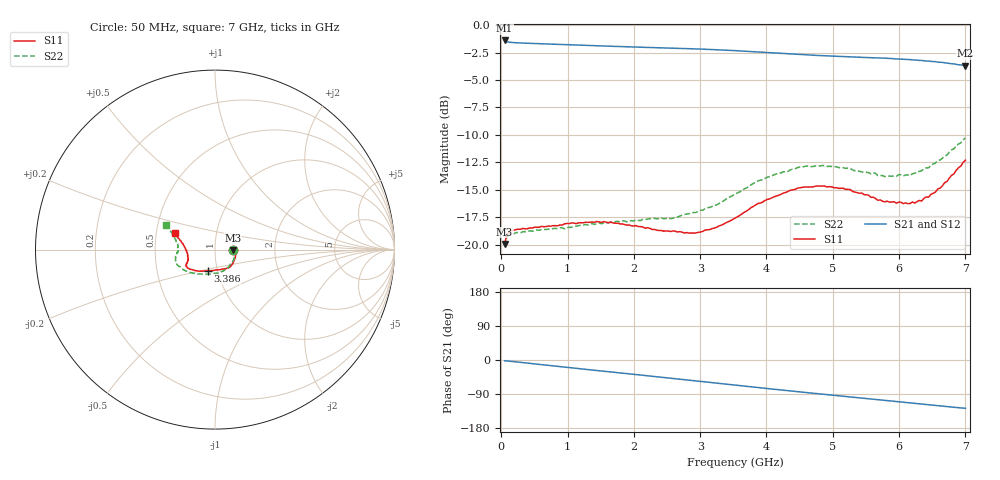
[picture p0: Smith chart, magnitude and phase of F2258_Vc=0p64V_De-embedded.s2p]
! Integrated Device Technology
! Corporate Headquarters
! 6024 Silver Creek Valley Road
! San Jose, CA 95138  USA
! Phone:  1-408-284-8200
! Toll Free:  1-800-223-1366
! Webpage:  http://www.idt.com/
! Timing and RF Division
! 515 Groton Road, Suite 102
! Westford, MA 01886-6024
! Device:  F2258
! Description: Voltage Variable RF Attenuator
! Frequency:  50.0 -  6000.00 MHz
! Package:  3x3 mm Thin QFN Plastic Package: 16 pin
! Ports:  2 RF, 2 DC
!  Pin  1  = NC
!  Pin  2  = NC
!  Pin  3  = RF2  = Port 2
!  Pin  4  = GND
!  Pin  5  = Vdd
!  Pin  6  = NC
!  Pin  7  = VCTRL
!  Pin  8  = NC
!  Pin  9  = GND
!  Pin 10  = RF1  = Port 1
!  Pin 11  = NC
!  Pin 12  = NC
!  Pin 13  = NC
!  Pin 14  = NC
!  Pin 15  = NC
!  Pin 16  = NC
! Vcntrl:  0.640 Volts
! Vdd:  +3.300 Volts
! Current:  1.113 mA
! Data:  The device was measured on a the F2258 evaluation board which has
!  individual transmission lines to the RF pins.  Data was collected
!  using a calibrated network analyzer.  The evaluation board was
!  de-embedded using a TRL calibration technique.
!  The reference plane is the edge of the package pin.
! Misc:  SN 10
!  Action Tracker AT0285
! Date Measured:  2014-12-10
! Date:  2016-01-13  MJV
! Note:
!  Integrated Device Technology supplies this data as a sample of measured
!  data at the package pin for this product.  Your particular data for this
!  product may vary.
!  Data was taken at 25 degrees C.
!  Integrated Device Technology reserves the right to change this data at anytime.
!Freq_(GHz)  S11M_(dB)  S11P_(deg)  S21M_(dB)  S21P_(deg)  S12M_(dB)  S12P_(deg)  S22M_(dB)  S22P_(deg)
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# GHz S dB R 50
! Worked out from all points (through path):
!   201 points, 50 MHz to 7 GHz, reference 50 ohm
!   highest |S21| = -1.40 dB at 50 MHz (marker M1); lowest = -3.7 dB at 7 GHz (marker M2)
!   group delay of S21, straight-line fit = 50.5 ps
!   lowest |S11| = -19.9 dB at 50 MHz (marker M3), VSWR 1.22, Z = 61.2 - j0.498 ohm
!   |S11| at or under -10 dB: start of sweep to end of sweep
!   |S22| runs from -20.1 to -10.3 dB; largest |S21 - S12| = 0.00097
!   S11 on the Smith chart (normalised r, x): 50 MHz: 1.22, -0.01; 3.386 GHz: 0.90, -0.22; 7 GHz: 0.62, +0.12
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0.05  -19.91 -2.3  -1.40 -2.0  -1.40 -2.0  -20.12 -2.7
0.08475  -19.06 -3.7  -1.51 -2.5  -1.51 -2.5  -19.31 -4.3
0.15425  -18.68 -6.0  -1.58 -3.7  -1.58 -3.7  -18.99 -7.5
0.71025  -18.28 -25.7  -1.72 -14.2  -1.72 -14.2  -18.57 -31.3
1.2315  -18.00 -42.8  -1.83 -23.9  -1.83 -23.9  -18.21 -53.0
1.6485  -17.92 -52.4  -1.93 -31.5  -1.92 -31.5  -17.94 -66.0
2.37825  -18.70 -68.7  -2.06 -44.8  -2.06 -44.8  -17.61 -85.3
2.58675  -18.73 -74.6  -2.10 -48.6  -2.10 -48.6  -17.59 -91.9
2.93425  -18.92 -88.4  -2.17 -55.1  -2.17 -55.1  -17.06 -104.3
3.386  -17.99 -109.3  -2.28 -63.7  -2.29 -63.7  -15.85 -122.7
3.525  -17.57 -115.3  -2.33 -66.3  -2.33 -66.3  -15.41 -127.9
4.0115  -15.87 -133.6  -2.50 -75.3  -2.50 -75.3  -13.84 -144.6
4.46325  -14.85 -144.1  -2.67 -83.5  -2.67 -83.5  -12.98 -156.5
4.7065  -14.72 -147.5  -2.74 -87.8  -2.75 -87.8  -12.87 -161.1
5.2625  -14.96 -153.8  -2.90 -97.4  -2.91 -97.4  -13.03 -169.9
5.64475  -15.78 -158.9  -2.99 -104.0  -2.99 -104.0  -13.49 -175.8
5.6795  -15.94 -158.8  -2.98 -104.6  -2.99 -104.6  -13.70 -176.0
5.85325  -16.11 -162.8  -3.04 -107.7  -3.05 -107.7  -13.74 179.3
6.166  -16.24 -171.0  -3.14 -113.3  -3.15 -113.2  -13.69 172.8
6.33975  -16.02 -178.4  -3.22 -116.3  -3.23 -116.3  -13.26 168.2
6.61775  -14.84 169.4  -3.38 -121.2  -3.39 -121.2  -12.28 161.3
7  -12.30 157.8  -3.70 -127.4  -3.71 -127.4  -10.27 153.3
